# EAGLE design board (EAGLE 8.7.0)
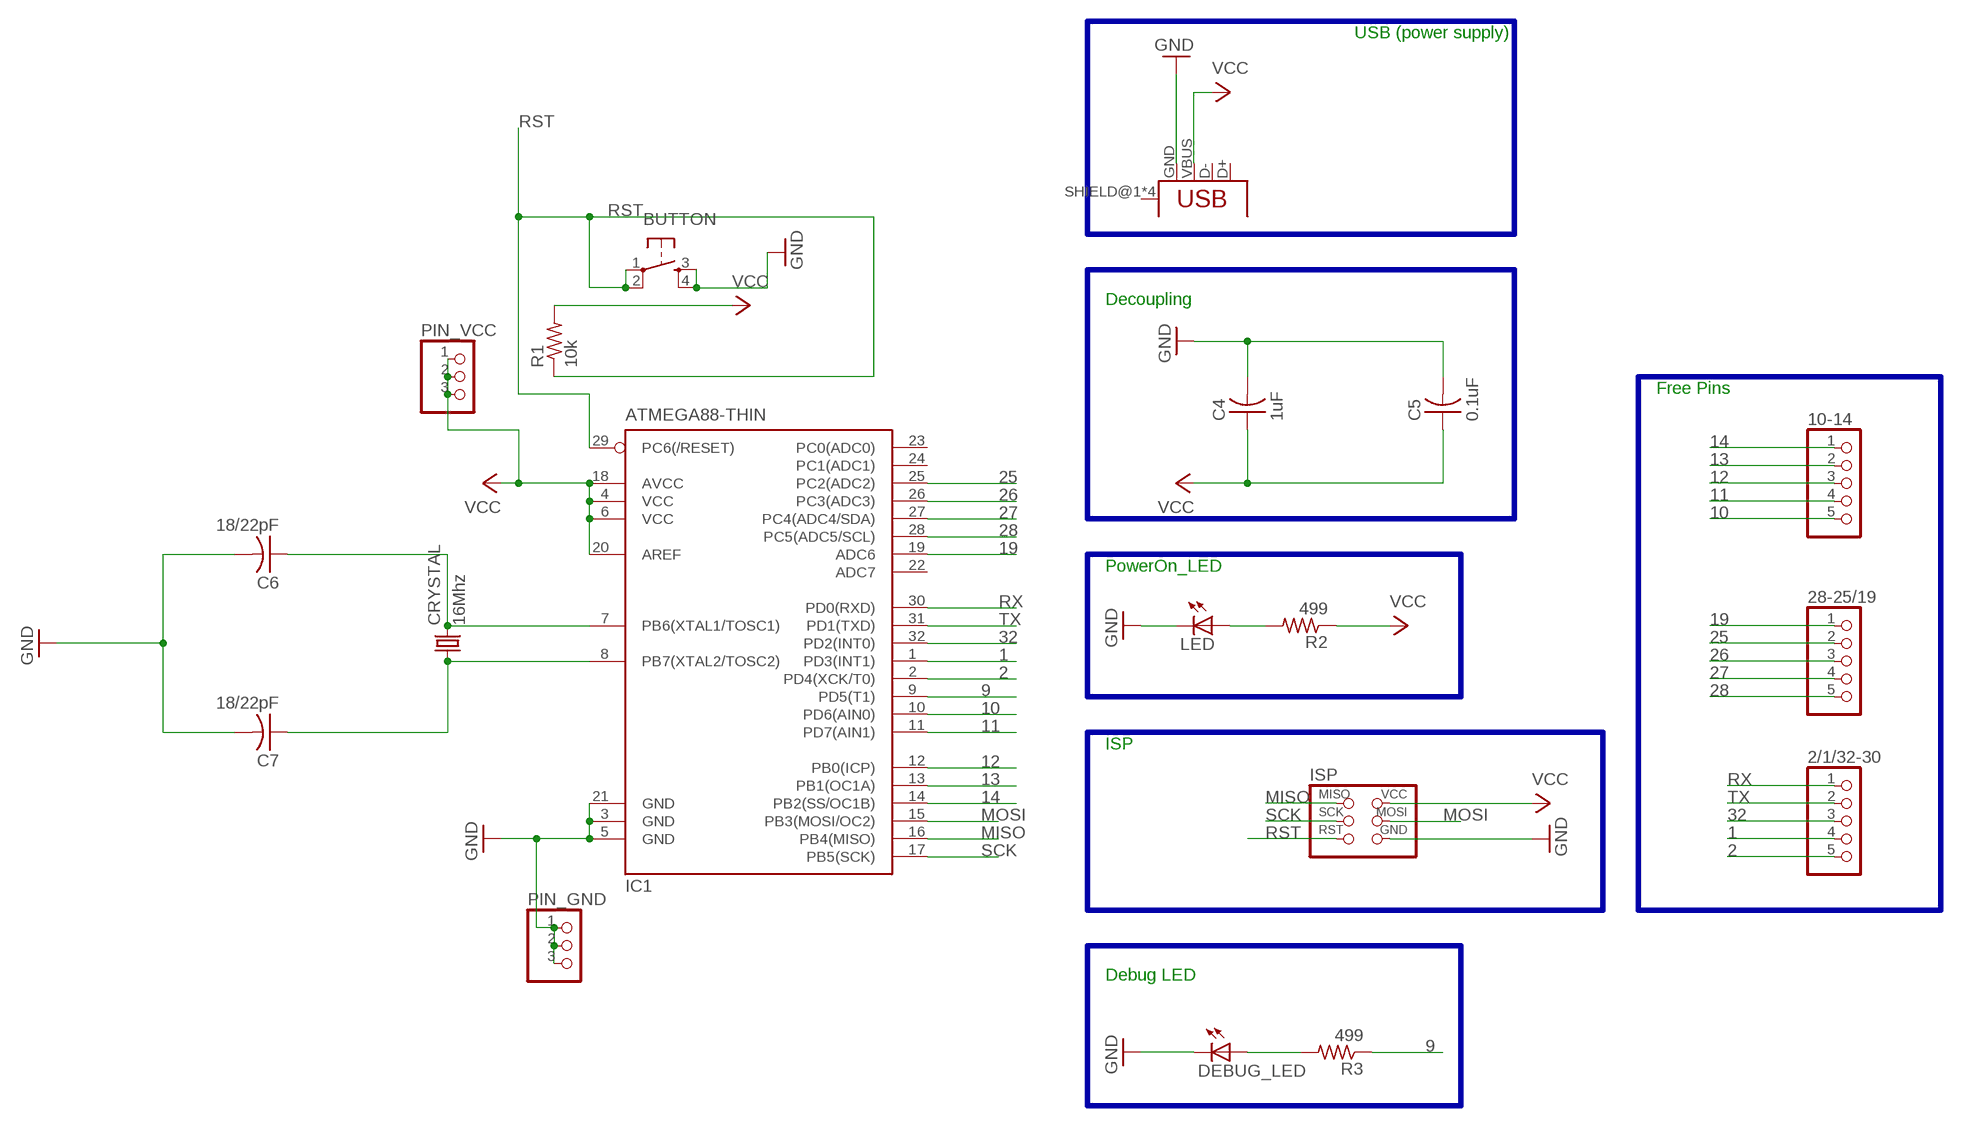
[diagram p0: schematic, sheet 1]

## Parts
2/1/32-30  PINHD-1X5  [1X05]
10-14  PINHD-1X5  [1X05]
28-25/19  PINHD-1X5  [1X05]
BUTTON  6MM_SWITCH6MM_SWITCH  [6MM_SWITCH]
C4  1uF  CAP-US1206FAB  [C1206FAB]
C5  0.1uF  CAP-US1206FAB  [C1206FAB]
C6  18/22pF  CAP-US1206FAB  [C1206FAB]
C7  18/22pF  CAP-US1206FAB  [C1206FAB]
CRYSTAL  16Mhz  CSM-7X-DU  [CSM-7X-DU]
DEBUG_LED  LEDFAB1206  [LED1206FAB]
IC1  ATMEGA88-THIN  [TQFP32-08THIN]
ISP  AVRISPSMD  [2X03SMD]
LED  LEDFAB1206  [LED1206FAB]
PIN_GND  PINHD-1X3  [1X03]
PIN_VCC  PINHD-1X3  [1X03]
R1  10k  RES-US1206FAB  [R1206FAB]
R2  499  RES-US1206FAB  [R1206FAB]
R3  499  RES-US1206FAB  [R1206FAB]
USB  USB_MINIB  [USB_MINIB]

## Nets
1: 2/1/32-30.4 IC1.1(PD3(INT1))
2: 2/1/32-30.5 IC1.2(PD4(XCK/T0))
9: IC1.9(PD5(T1)) R3.1
10: 10-14.5 IC1.10(PD6(AIN0))
11: 10-14.4 IC1.11(PD7(AIN1))
12: 10-14.3 IC1.12(PB0(ICP))
13: 10-14.2 IC1.13(PB1(OC1A))
14: 10-14.1 IC1.14(PB2(SS/OC1B))
19: 28-25/19.1 IC1.19(ADC6)
25: 28-25/19.2 IC1.25(PC2(ADC2))
26: 28-25/19.3 IC1.26(PC3(ADC3))
27: 28-25/19.4 IC1.27(PC4(ADC4/SDA))
28: 28-25/19.5 IC1.28(PC5(ADC5/SCL))
32: 2/1/32-30.3 IC1.32(PD2(INT0))
GND: BUTTON.3(S) BUTTON.4(S1) C4.2 C5.2 C6.2 C7.2 DEBUG_LED.2(C) IC1.3(GND) IC1.5(GND) IC1.21(GND) ISP.6(GND) LED.2(C) PIN_GND.1 PIN_GND.2 PIN_GND.3 USB.GND
MISO: IC1.16(PB4(MISO)) ISP.1(MISO)
MOSI: IC1.15(PB3(MOSI/OC2)) ISP.4(MOSI)
N$3: LED.1(A) R2.2
N$4: DEBUG_LED.1(A) R3.2
N$5: C7.1 CRYSTAL.1 IC1.8(PB7(XTAL2/TOSC2))
N$6: C6.1 CRYSTAL.2 IC1.7(PB6(XTAL1/TOSC1))
RST: BUTTON.1(P) BUTTON.2(P1) IC1.29(PC6(/RESET)) ISP.5(RST) R1.1
RX: 2/1/32-30.1 IC1.30(PD0(RXD))
SCK: IC1.17(PB5(SCK)) ISP.3(SCK)
TX: 2/1/32-30.2 IC1.31(PD1(TXD))
VCC: C4.1 C5.1 IC1.4(VCC) IC1.6(VCC) IC1.18(AVCC) IC1.20(AREF) ISP.2(VCC) PIN_VCC.1 PIN_VCC.2 PIN_VCC.3 R1.2 R2.1 USB.VBUS
Unconnected: IC1.22(ADC7) IC1.23(PC0(ADC0)) IC1.24(PC1(ADC1)) USB.D+ USB.D- USB.SHIELD@1(SHIELD) USB.SHIELD@2(SHIELD) USB.SHIELD@3(SHIELD) USB.SHIELD@4(SHIELD)

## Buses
B$1
B$2
B$5
B$6
B$7
B$3

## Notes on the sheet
- USB (power supply)
- Decoupling
- Free Pins
- PowerOn_LED
- ISP
- Debug LED

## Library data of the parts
2/1/32-30 10-14 28-25/19 = pinhead:PINHD-1X5: PIN HEADER
BUTTON = 1_fab:6MM_SWITCH: OMRON SWITCH
C4-C7 = 1_fab:CAP-US
CRYSTAL = crystal:CSM-7X-DU: SMD CRYSTAL; OC_FARNELL: unknown; OC_NEWARK: unknown
DEBUG_LED LED = 1_fab:LED: LED
IC1 = 1_fab:ATMEGA88-THIN
ISP = 1_fab:AVRISP
PIN_GND PIN_VCC = pinhead:PINHD-1X3: PIN HEADER
R1-R3 = 1_fab:RES-US: Resistor (US Symbol)
USB = 1_fab:USB_MINIB

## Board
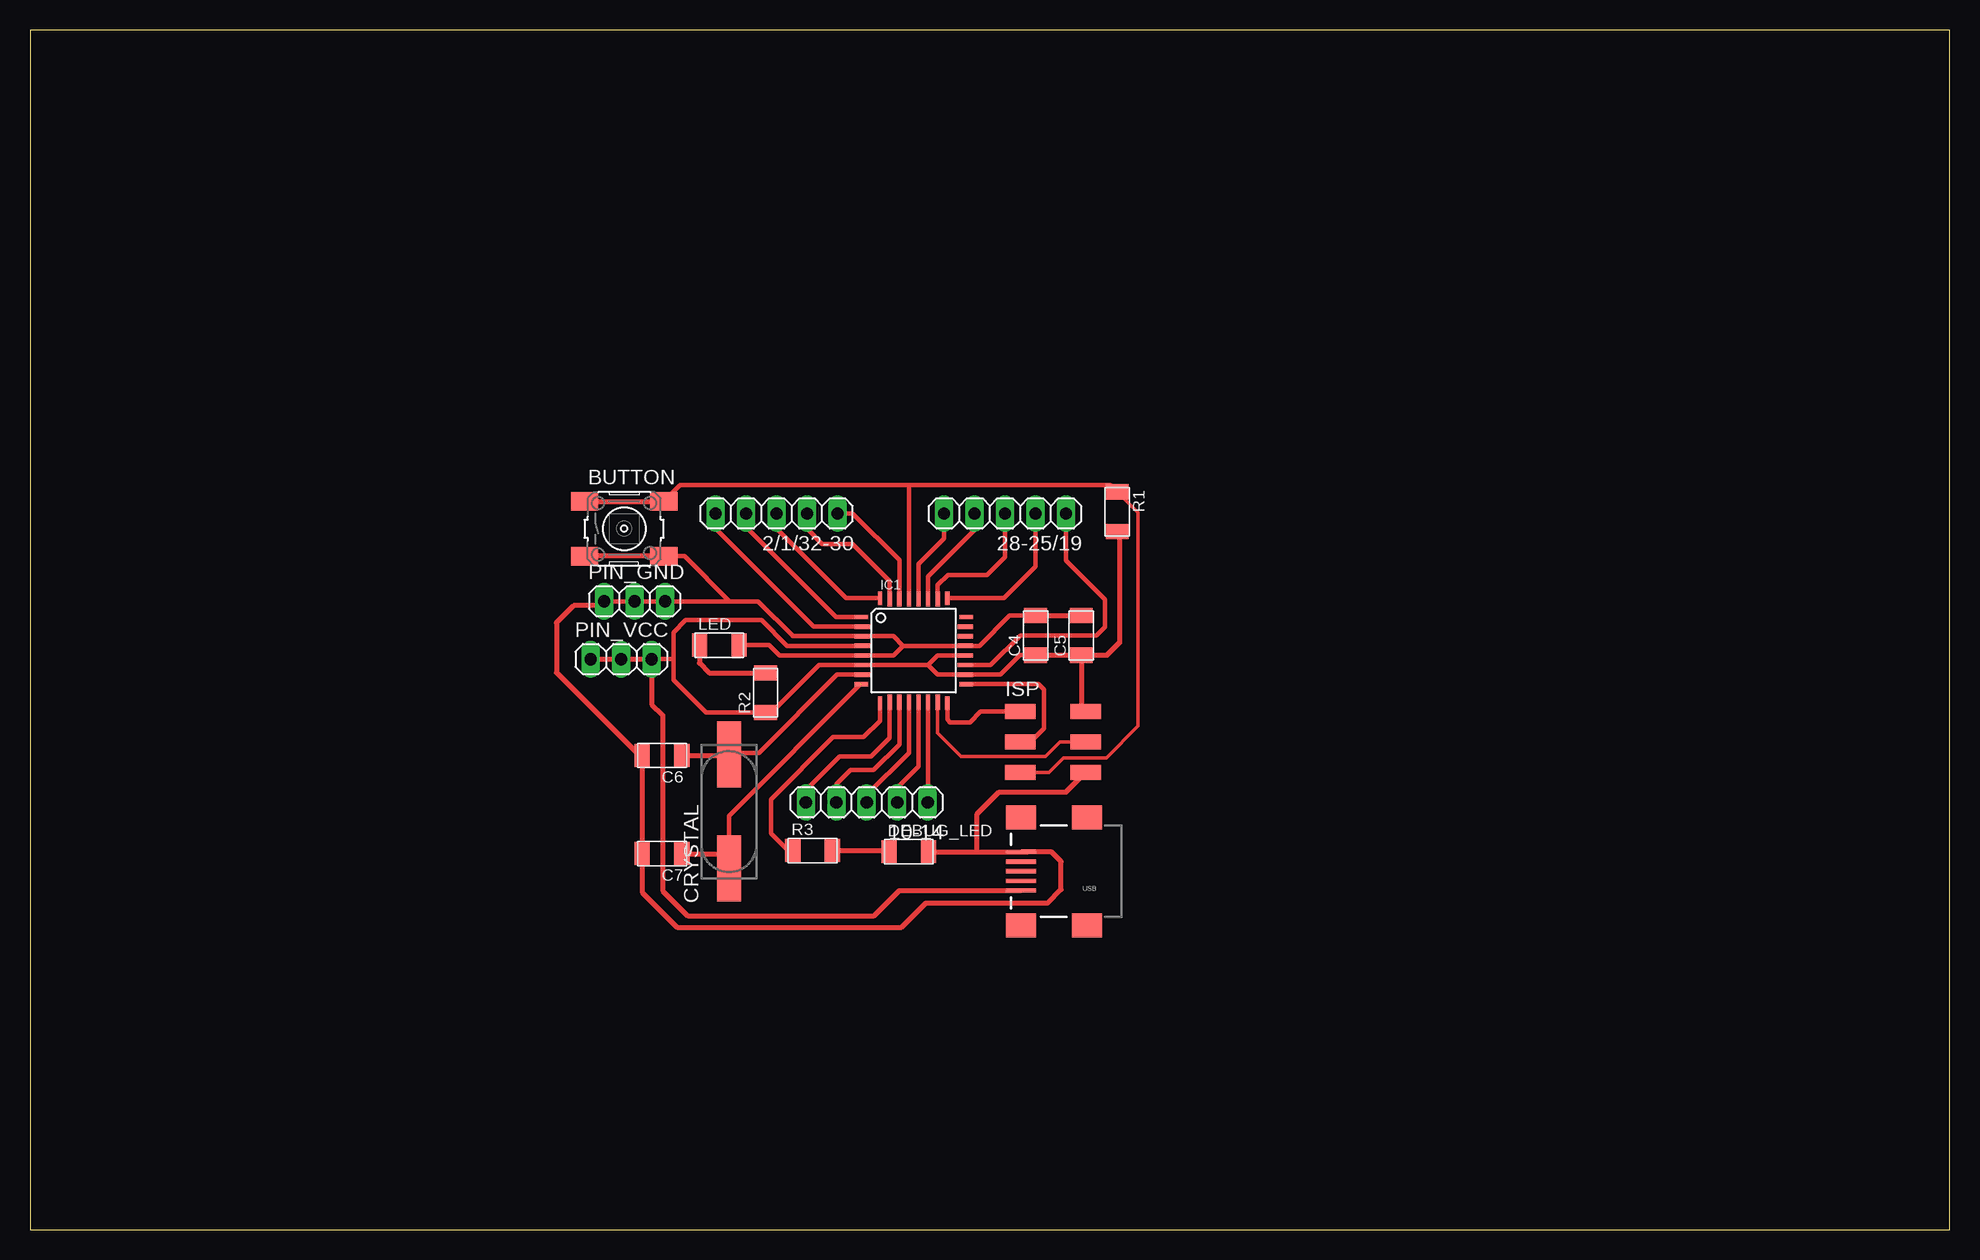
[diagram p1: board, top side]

Size 160 x 100 mm. Coordinates in mm from the lower left corner, seen from the top.
Outline: 0,0 160,0 160,100 0,100 0,0
Copper layers (1*16): Top 0.035mm / dielectric 1.5mm / Bottom 0.035mm
Design rules "default": minimum track width 6mil, minimum drill 0.35mm, track to track 6mil, track to pad 6mil, pad to pad 6mil, via to via 6mil, smd to smd 6mil, copper to edge 40mil, drill to drill 6mil, minimum pad ring 10mil, minimum via ring 8mil, stop-mask expansion 4mil, vias tented up to drill 0mil, thermal gap 10mil

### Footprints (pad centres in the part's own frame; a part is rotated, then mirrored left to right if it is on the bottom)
1X05 = drill 1.016 long: 1 -5.08,0; 2 -2.54,0; 3 0,0; 4 2.54,0; 5 5.08,0
6MM_SWITCH = smd 2.286 x 1.524: 1 -3.302,2.286; 2 3.302,2.286; 3 -3.302,-2.286; 4 3.302,-2.286
C1206FAB = smd 1.27 x 1.905: 1 -1.651,0; 2 1.651,0
CSM-7X-DU = smd 5.5 x 2: 1 -4.75,0; 2 4.75,0
LED1206FAB = smd 1.27 x 1.905: 1 -1.651,0; 2 1.651,0
TQFP32-08THIN = smd 1.118 x 0.356: 1 -4.369,2.8; 8 -4.369,-2.8; 17 4.369,-2.8; 24 4.369,2.8 | smd 1.27 x 0.356: 2 -4.293,2; 3 -4.293,1.2; 4 -4.293,0.4; 5 -4.293,-0.4; 6 -4.293,-1.2; 7 -4.293,-2; 18 4.293,-2; 19 4.293,-1.2; 20 4.293,-0.4; 21 4.293,0.4; 22 4.293,1.2; 23 4.293,2 | smd 0.356 x 1.118: 9 -2.8,-4.369; 16 2.8,-4.369; 25 2.8,4.369; 32 -2.8,4.369 | smd 0.356 x 1.27: 10 -2,-4.293; 14 1.2,-4.293; 15 2,-4.293; 26 2,4.293; 27 1.2,4.293; 31 -2,4.293 | smd 0.35 x 1.27: 11 -1.2,-4.293; 12 -0.4,-4.293; 13 0.4,-4.293; 28 0.4,4.293; 29 -0.4,4.293; 30 -1.2,4.293
2X03SMD = smd 2.54 x 1.27: 1 -2.54,2.54; 2 2.92,2.54; 3 -2.54,0; 4 2.92,0; 5 -2.54,-2.54; 6 2.92,-2.54
1X03 = drill 1.016 long: 1 -2.54,0; 2 0,0; 3 2.54,0
R1206FAB = smd 1.27 x 1.905: 1 -1.651,0; 2 1.651,0
USB_MINIB = smd 2.5 x 0.35: D+ 3.77,0; D- 3.77,0.8; GND 3.77,-1.6; ID 3.77,-0.8; VBUS 3.77,1.6 | smd 2.5 x 2: SHIELD@1 -1.73,-4.5; SHIELD@2 -1.73,4.5; SHIELD@3 3.77,4.5; SHIELD@4 3.77,-4.5

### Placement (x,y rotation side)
2/1/32-30  62.23,59.69 180 top
10-14  69.75,35.61 180 top
28-25/19  81.28,59.69 180 top
BUTTON  49.53,58.42 0 top
C4  83.82,49.53 90 top
C5  87.63,49.53 90 top
C6  52.68,39.52 180 top
C7  52.68,31.34 180 top
CRYSTAL  58.27,34.85 90 top
DEBUG_LED  73.25,31.5 0 top
IC1  73.66,48.26 0 top
ISP  85.09,40.64 0 top
LED  57.45,48.72 0 top
PIN_GND  50.39,52.37 0 top
PIN_VCC  49.28,47.55 0 top
R1  90.63,59.84 270 top
R2  61.32,44.75 90 top
R3  65.23,31.6 0 top
USB  86.36,29.87 180 top

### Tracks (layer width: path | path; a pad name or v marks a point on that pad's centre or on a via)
1
  Top 0.356: IC1.1 67.2,51.06 59.69,58.57 2/1/32-30.4
2
  Top 0.356: IC1.2 65.31,50.26 57.15,58.42 2/1/32-30.5
9
  Top 0.356: IC1.9 70.86,42.41 69.49,41.05 66.95,41.05 61.77,35.87 61.77,33.02 63.2,31.6 R3.1
10
  Top 0.356: IC1.10 71.66,40.98 70.1,39.42 67.46,39.42 64.67,36.63 10-14.5
11
  Top 0.356: IC1.11 72.46,40.46 70.31,38.3 68.38,38.3 67.21,37.13 10-14.4
12
  Top 0.356: IC1.12 73.25,39.73 69.75,36.22 10-14.3
13
  Top 0.356: IC1.13 74.06,38.6 72.29,36.83 10-14.2
14
  Top 0.356: IC1.14 74.86,35.64 10-14.1
19
  Top 0.356: IC1.19 80.08,47.06 82.55,49.53 88.9,49.53 89.61,50.24 89.61,51.61 89.61,51.82 89.61,52.53 86.36,55.78 28-25/19.1
25
  Top 0.356: IC1.25 81.18,52.63 83.82,55.27 28-25/19.2
26
  Top 0.356: 75.69,52.59 IC1.26 75.66,53.71 76.5,54.56 79.76,54.56 81.28,56.08 28-25/19.3
27
  Top 0.356: IC1.27 74.86,54.44 78.74,58.32 28-25/19.4
28
  Top 0.356: IC1.28 74.06,55.47 76.2,57.61 28-25/19.5
32
  Top 0.356: IC1.32 68.02,52.63 62.23,58.42 2/1/32-30.3
GND
  Top 0.356: 72.79,48.66 IC1.21 79.14,48.66 81.66,51.18 C4.2 | 72.79,48.66 71.99,47.86 IC1.5 62.48,47.86 61.62,48.72 LED.2 | 72.79,48.66 71.99,49.46 IC1.3 63.6,49.46 | 63.6,49.46 63.57,49.46 | 58.32,52.38 PIN_GND.3 PIN_GND.2 PIN_GND.1 47.5,52.02 | 58.32,52.38 60.69,52.38 63.6,49.46 | BUTTON.4 54.56,56.13 58.32,52.38
  Top 0.406: 88.39,37.72 ISP.6 | C4.2 C5.2 | BUTTON.4 BUTTON.3 46.23,55.83 | 88.09,38.02 ISP.6 | 51.03,31.45 C7.2 | 47.5,52.02 45.31,52.02 43.89,50.6 43.89,46.43 51,39.32 51.03,39.32 C6.2 C7.2 | 83.11,31.47 85.17,31.47 85.95,30.68 85.95,28.35 84.84,27.23 74.68,27.23 72.64,25.2 53.95,25.2 51.03,28.12 C7.2 | 83.11,31.47 USB.GND | DEBUG_LED.2 78.94,31.5 | 78.94,31.5 83.08,31.5 83.11,31.47 | 78.94,31.5 78.94,34.65 80.77,36.47 86.36,36.47 87.99,38.1 ISP.6
MISO
  Top 0.356: IC1.16 76.46,42.51 76.71,42.27 78.33,42.27 79.25,43.18 ISP.1
MOSI
  Top 0.305: IC1.15 75.66,41.38 77.62,39.42 84.63,39.42 85.85,40.64 ISP.4
N$3
  Top 0.406: 55.78,48.69 LED.1 55.8,47.22 56.62,46.41 R2.2
N$4
  Top 0.406: R3.2 71.5,31.6 DEBUG_LED.1
N$5  (1 unrouted)
  Top 0.356: CRYSTAL.1 58.27,31.29 58.27,34.49 69.23,45.46
  Top 0.406: C7.1 54.38,31.29 58.27,31.29
N$6
  Top 0.356: CRYSTAL.2 58.39,39.73 60.76,39.73 67.29,46.26 IC1.7
  Top 0.406: C6.1 58.32,39.52 58.4,39.6 | 58.73,39.93 58.4,39.6 | 58.4,39.6 CRYSTAL.2
RST
  Top 0.305: ISP.5 84.94,38.1 86.16,39.32 89.71,39.32 92.35,41.96 92.35,59.77 R1.1
  Top 0.356: ISP.5 83.62,38.1 | IC1.29 73.26,62.08 | BUTTON.2 54.2,62.08 73.26,62.08 | R1.1 90.04,62.08 73.26,62.08
  Top 0.406: BUTTON.1 BUTTON.2
RX
  Top 0.356: 2/1/32-30.1 68.58,59.69 72.46,55.81 IC1.30
SCK
  Top 0.356: IC1.17 84.08,45.46 84.53,45.01 84.53,41.76 83.41,40.64 ISP.3
TX
  Top 0.356: 2/1/32-30.2 64.77,58.42 66.04,57.15 68.58,57.15 71.12,54.61 71.54,54.19 | 71.66,54.07 71.54,54.19 | 71.54,54.19 arc-45 71.66,53.9 IC1.31
VCC
  Top 0.356: 74.86,47.06 IC1.6 65.75,47.06 61.8,43.1 R2.1 56.34,43.1 53.65,45.8 53.65,47.55 | 74.86,47.06 75.66,46.26 IC1.18 80.91,46.26 82.53,47.88 C4.1 | 74.86,47.06 75.66,47.86 IC1.20 | 53.65,47.55 53.65,49.78 54.66,50.8 60.96,50.8 63.1,48.66 IC1.4 | PIN_VCC.3 53.65,47.55
  Top 0.406: C4.1 C5.1 | C5.1 89.79,47.88 90.83,48.92 90.83,57.99 R1.2 | C5.1 87.63,43.56 ISP.2 | PIN_VCC.1 PIN_VCC.2 PIN_VCC.3 51.82,43.79 52.73,42.88 52.73,28.25 54.81,26.16 70.36,26.16 72.47,28.27 USB.VBUS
